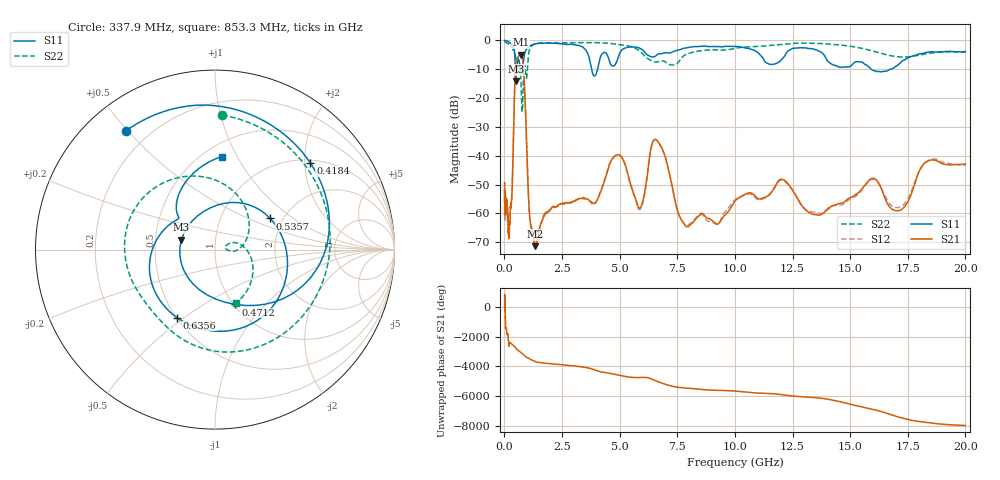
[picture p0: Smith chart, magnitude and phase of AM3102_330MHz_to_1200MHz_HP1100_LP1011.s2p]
! Date/Time: Tue, Sep 11, 2018 5:21 PM
! Network Analyzer: Agilent Technologies E8362B Rev: A.07.50.63
! Sweep from 0.010 to 20.000 GHz, 1601 Points, Sweep Type: LOG
! Power Supply: 4.949 V, 0.001 A
# Hz S DB R 50
!freq MagS11 AngS11 MagS21 AngS21 MagS12 AngS12 MagS22 AngS22
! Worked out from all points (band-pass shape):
!   1601 points, 10 MHz to 20 GHz, reference 50 ohm
!   highest |S21| = -4.95 dB at 709 MHz (marker M1); lowest = -71.4 dB at 1.346 GHz (marker M2)
!   |S21| within 3 dB of the highest: 489.7 MHz to 809.4 MHz (319.7 MHz wide, 49.2 % of centre)
!   lowest |S11| = -14.2 dB at 496.5 MHz (marker M3), VSWR 1.48, Z = 34.1 + j3.96 ohm
!   |S11| at or under -10 dB: 706.7 MHz to 794.7 MHz (87.94 MHz wide, 11.7 % of centre); 3.787 GHz to 4.044 GHz (257.1 MHz wide, 6.57 % of centre); 15.91 GHz to 16.77 GHz (861.4 MHz wide, 5.27 % of centre)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
!   |S22| runs from -24.8 to -0.2 dB; largest |S21 - S12| = 0.0096
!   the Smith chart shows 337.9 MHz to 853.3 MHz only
!   S11 on the Smith chart (normalised r, x): 337.9 MHz: 0.12, +0.50; 418.4 MHz: 1.07, +2.13; 471.2 MHz: 1.02, -0.69; 535.7 MHz: 1.72, +0.68; 635.6 MHz: 0.50, -0.47; 853.3 MHz: 0.61, +0.87
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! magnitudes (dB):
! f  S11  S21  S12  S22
! 10 MHz  0.0  -49.6  -56.3  -0.2
! 35.55 MHz  -0.1  -58.2  -59.3  -0.5
! 126.4 MHz  -0.3  -57.6  -58.4  -1.0
! 192 MHz  -0.5  -68.8  -66.6  -1.2
! 337.9 MHz  -1.6  -51.6  -51.5  -2.5
! 418.4 MHz  -2.9  -24.6  -24.7  -4.1
! 447.2 MHz  -4.6  -16.1  -16.1  -4.6
! 471.2 MHz  -9.7  -10.6  -10.6  -5.4
! 496.5 MHz  -14.2  -7.4  -7.4  -6.2
! 535.7 MHz  -9.0  -6.2  -6.2  -6.0
! 635.6 MHz  -7.2  -5.3  -5.4  -7.4
! 709 MHz  -10.1  -4.9  -5.0  -12.9
! 853.3 MHz  -5.7  -12.8  -13.0  -9.9
! 1.087 GHz  -2.1  -60.2  -60.4  -3.3
! 1.346 GHz  -1.2  -71.4  -70.3  -1.2
! 1.59 GHz  -1.0  -63.3  -63.8  -1.0
! 3.902 GHz  -12.3  -56.5  -56.8  -0.8
! 4.878 GHz  -7.3  -39.8  -39.8  -1.4
! 5.652 GHz  -2.3  -54.1  -54.4  -2.6
! 6.58 GHz  -5.3  -34.4  -34.6  -7.5
! 7.958 GHz  -2.5  -64.7  -64.1  -4.6
! 20 GHz  -3.9  -42.9  -43.4  -4.1
